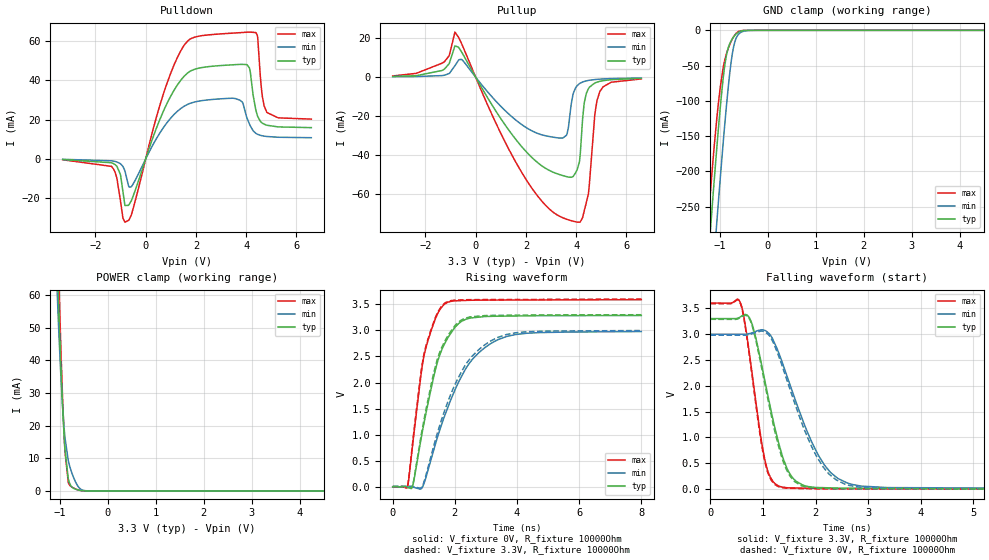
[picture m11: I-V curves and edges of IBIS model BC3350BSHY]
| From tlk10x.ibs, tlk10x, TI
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|   Model
[Model]   BC3350BSHY
Model_type   I/O
Polarity   Non-Inverting
Enable   Active-Low
Vinl = 0.99
Vinh = 2.31
Vmeas = 1.65
Vref = 1.65
Cref = 1pF
Rref = 10000
|   typ   min   max
C_comp   1.892pF   1.852pF   1.956pF
[Voltage Range]   3.3   3   3.6
[Temperature Range]   25   125   -40
[Pullup Reference]   3.3   3   3.6
[Pulldown Reference]   -0   -0   -0
[Power Clamp Reference]   3.3   3   3.6
[GND Clamp Reference]   -0   -0   -0
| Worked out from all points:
|   slope of the pulldown table from 0 to 0.495 V, typ, clamps not added: 27.8 ohm
|   slope of the pullup table from 0 to 0.495 V, typ, clamps not added: 45 ohm
|   GND clamp passes 1 mA (typ) near -0.55 V on its own axis
|   POWER clamp passes 1 mA (typ) near -0.73 V on its own axis
|   falling waveform, V_fixture 3.3V, R_fixture 10000Ohm: 20-80 % time 436ps typ, 697ps min, 300ps max; typ from 3.3 V to 0.008 V
|   rising waveform, V_fixture 0V, R_fixture 10000Ohm: 20-80 % time 744ps typ, 1.22ns min, 545ps max; typ from 0 V to 3.29 V
|   rising waveform, V_fixture 3.3V, R_fixture 10000Ohm: 20-80 % time 729ps typ, 1.17ns min, 542ps max; typ from 0.008 V to 3.3 V
|   falling waveform, V_fixture 0V, R_fixture 10000Ohm: 20-80 % time 428ps typ, 678ps min, 296ps max; typ from 3.29 V to 0 V
[Pulldown]
|   Voltage   I(typ)   I(min)   I(max)
-3.3V     -306.9uA   -177.2uA   -405.8uA
-1.36V    -1.92mA    -935.1uA   -3.756mA
-904.2mV  -16.59mA   -3.768mA   -30.06mA
-676.5mV  -23.41mA   -13.77mA   -31.09mA
976.8mV   31.4mA     20.44mA    42.88mA
2.224V    46.37mA    29.58mA    62.55mA
3.749V    47.99mA    29.83mA    64.09mA
4.036V    47.8mA     20.63mA    64.34mA
4.392V    24.4mA     12.94mA    64.04mA
4.64V     18.21mA    11.76mA    31.97mA
4.818V    17.14mA    11.41mA    23.72mA
6.59V     15.9mA     10.79mA    20.22mA
[GND Clamp]
|   Voltage   I(typ)   I(min)   I(max)
-3.3V     -2.327A    -2.431A    -2.267A
-1.251V   -331.9mA   -441.7mA   -275.1mA
-1.142V   -233.8mA   -342.1mA   -183mA
-1.063V   -165.7mA   -271.4mA   -124mA
-993.3mV  -110.6mA   -211.3mA   -81.81mA
-933.9mV  -69.63mA   -161.9mA   -54.3mA
-864.6mV  -35.68mA   -108.2mA   -33.39mA
-795.3mV  -19.12mA   -61.61mA   -20.33mA
-735.9mV  -11.5mA    -31.56mA   -11.69mA
-676.5mV  -6.245mA   -13.89mA   -5.434mA
-597.3mV  -2.105mA   -4.642mA   -1.279mA
6.59V     0A         0A         0A
[Pullup]
|   Voltage   I(typ)   I(min)   I(max)
-3.3V     399.3uA    220.7uA    635.9uA
-1.251V   4.082mA    981.5uA    7.893mA
-825mV    16.09mA    5.869mA    23.18mA
1.531V    -30.93mA   -21.37mA   -42.19mA
3.214V    -49.55mA   -31.12mA   -70.63mA
3.62V     -51.15mA   -29.63mA   -73.08mA
3.868V    -51.13mA   -9.191mA   -74.04mA
4.125V    -43.72mA   -3.369mA   -74.58mA
4.402V    -8.366mA   -1.906mA   -64.53mA
4.749V    -2.95mA    -1.219mA   -18.38mA
4.937V    -2.145mA   -1.017mA   -7.52mA
6.59V     -611.8uA   -409.7uA   -889.8uA
[POWER Clamp]
|   Voltage   I(typ)   I(min)   I(max)
-3.3V     1.546A     1.464A     1.615A
-1.053V   70.2mA     59.69mA    81.95mA
-1.023V   56.52mA    49.07mA    65.63mA
-1.013V   52.21mA    45.75mA    60.42mA
-943.8mV  26.09mA    25.94mA    28.48mA
-894.3mV  12.77mA    16.41mA    12.16mA
-825mV    3.748mA    9.344mA    2.589mA
-775.5mV  1.705mA    6.627mA    1.452mA
-686.4mV  612.2uA    3.169mA    684.3uA
-567.6mV  145.8uA    561.8uA    126.2uA
-409.2mV  4.012uA    20.73uA    1.375uA
6.59V     0A         0A         0A
[Ramp]
R_load = 10000
|   typ   min   max
dV/dt_r   1.97127/7.44347e-10   1.78611/1.21613e-09   2.15306/5.44771e-10
dV/dt_f   1.97486/4.35675e-10   1.79076/6.94866e-10   2.15599/2.98812e-10
[Falling Waveform]
V_fixture = 3.3V
V_fixture_min = 3V
V_fixture_max = 3.6V
R_fixture = 10000Ohm
C_fixture = 0F
|   Time   V(typ)   V(min)   V(max)
0s        3.3V       2.997V     3.6V
576.4ps   3.335V     2.997V     3.597V
797.2ps   3.189V     3.025V     2.221V
1.029ns   2.137V     3.072V     607.5mV
1.288ns   935.8mV    2.669V     67.28mV
1.459ns   399.5mV    2.184V     27.92mV
1.633ns   151.3mV    1.676V     22.4mV
2.168ns   28.45mV    468.1mV    13.12mV
2.599ns   19.01mV    121.4mV    10.66mV
8ns       8.339mV    12.34mV    6.674mV
[Rising Waveform]
V_fixture = 0V
V_fixture_min = 0V
V_fixture_max = 0V
R_fixture = 10000Ohm
C_fixture = 0F
|   Time   V(typ)   V(min)   V(max)
0s        39.32uV    689uV      381.9nV
459.3ps   -3.57mV    1.636mV    -17.09mV
625.8ps   -12.06mV   1.979mV    724.5mV
907.4ps   905.3mV    -37.85mV   2.132V
1.029ns   1.29V      104.5mV    2.571V
1.385ns   2.272V     842.8mV    3.239V
1.671ns   2.745V     1.362V     3.505V
2.441ns   3.228V     2.349V     3.576V
3.375ns   3.271V     2.82V      3.581V
8ns       3.285V     2.978V     3.588V
[Rising Waveform]
V_fixture = 3.3V
V_fixture_min = 3V
V_fixture_max = 3.6V
R_fixture = 10000Ohm
C_fixture = 0F
|   Time   V(typ)   V(min)   V(max)
0s        8.338mV    12.34mV    6.674mV
472.8ps   1.655mV    13.18mV    6.986mV
625.8ps   2.256mV    13.45mV    764.5mV
907.4ps   961.6mV    -18.35mV   2.186V
1.018ns   1.322V     119.9mV    2.576V
1.418ns   2.408V     993.6mV    3.307V
1.671ns   2.788V     1.462V     3.522V
2.404ns   3.245V     2.394V     3.588V
3.375ns   3.288V     2.864V     3.591V
8ns       3.3V       2.997V     3.6V
[Falling Waveform]
|Gnd
V_fixture = 0V
V_fixture_min = 0V
V_fixture_max = 0V
R_fixture = 10000Ohm
C_fixture = 0F
|   Time   V(typ)   V(min)   V(max)
0s        3.285V     2.978V     3.588V
576.4ps   3.323V     2.978V     3.581V
769.7ps   3.237V     2.996V     2.383V
1.018ns   2.129V     3.05V      615.6mV
1.131ns   1.565V     2.957V     224.6mV
1.288ns   868.7mV    2.606V     52.02mV
1.517ns   248.7mV    1.925V     15.52mV
2ns       19.06mV    673.8mV    6.933mV
2.551ns   9.881mV    100.3mV    4.405mV
8ns       40.11uV    687.2uV    860.5nV
